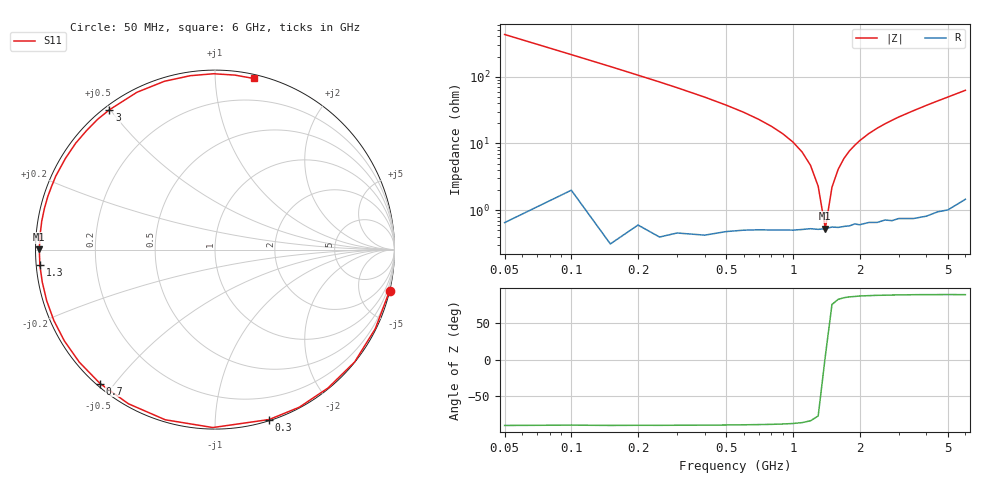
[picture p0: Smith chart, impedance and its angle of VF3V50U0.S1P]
! Infineon Technologies  Discrete & RF Semiconductors
! BBY 58-03
! Si Tuning Diode in SOD323
! VR = 3.5 V
! S-Parameters:  June  1999
# GHz  S  MA  R  50
!  f  S11
! GHz  MAG  ANG
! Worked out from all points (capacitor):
!   34 points, 50 MHz to 6 GHz, reference 50 ohm
!   read as one part to ground: C = 7.4 pF near 50 MHz
!   lowest |Z| = 532 mohm at 1.4 GHz (marker M1)
!   series resonance near 1.398 GHz, so ESL is about 1.8 nH
!   S11 on the Smith chart (normalised r, x): 50 MHz: 0.01, -8.58; 300 MHz: 0.01, -1.37; 700 MHz: 0.01, -0.46; 1.3 GHz: 0.01, -0.04; 3 GHz: 0.02, +0.50; 6 GHz: 0.03, +1.25
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0.05  0.9997 -13.3
0.1  0.9959 -26.3
0.15  0.9986 -38.8
0.2  0.9956 -50.8
0.25  0.9958 -61.9
0.3  0.9937 -72.3
0.4  0.9915 -90.7
0.5  0.9878 -106.3
0.6  0.9851 -119.3
0.7  0.9833 -130.6
0.8  0.9822 -140.3
0.9  0.9814 -148.8
1  0.9809 -156.3
1.1  0.98 -163.1
1.3  0.9796 -174.9
1.4  0.979 179.9
1.6  0.9783 170.7
1.8  0.9774 162.4
2  0.9771 155.2
2.4  0.9767 142.6
2.8  0.9769 132.0
3  0.9762 127.1
3.5  0.9785 116.4
4  0.9792 106.7
4.5  0.9786 98.1
5  0.9798 90.5
5.5  0.9785 83.5
6  0.9775 77.3
